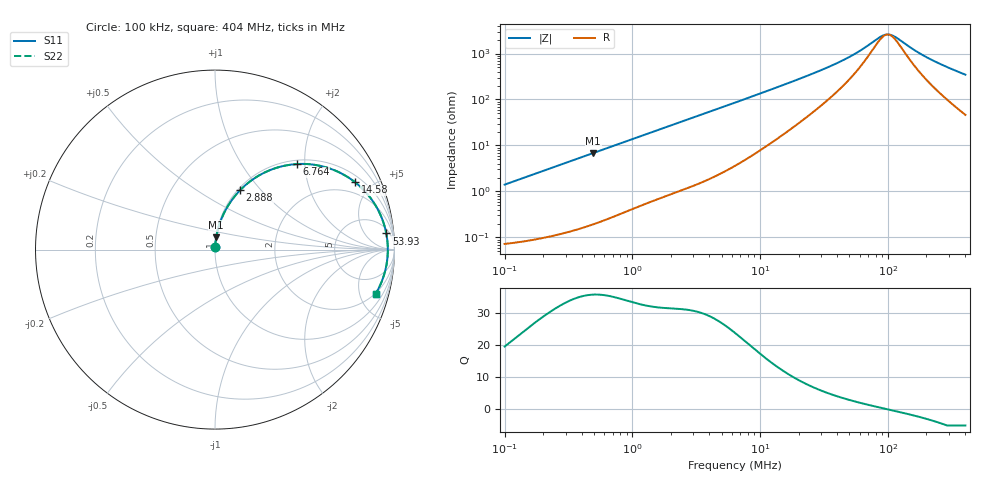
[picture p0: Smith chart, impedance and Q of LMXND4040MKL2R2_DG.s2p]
! LMXND4040MKL2R2_DG  S-PARAMETER MODEL  ( General Type )
! Model Generated by TAIYO YUDEN Corporation (http://www.ty-top.com)
! Version 1.0
! TAIYO YUDEN Control No. 191023NI43SB-FBB
! Copyright(c) 2019 TAIYO YUDEN CO.,LTD. All Rights Reserved.
! Product Description (link to TY-COMPAS)
! https://ds.yuden.co.jp/TYCOMPAS/or/detail?pn=LMXND4040MKL2R2MDG&u=M
! Products Name : Inductors
! Characteristics :
!  Inductance : 2.2 uH , SRF(min) : 70 MHz , DC Resistance(max) : 0.072 Ohm
!  Rated Current : Saturation :1650 mA , Temp Rise : 1900 mA
!  Case Size : 4.0 x 4.0 / 0.157 x 0.157 [mm/inch] , Thickness : 1.2 / 0.047 [mm/inch]
!  (Conditions: Temperature = 25 degC , DC Bias Current/Voltage = 0A / 0V)
! External Node Assignments :
!  1  o---GGG---o  2
! GND o---------o GND
! Frequency Range : 0.1MHz  -  403.964729MHz  [ 402 STEP ]
# MHz S RI R 50
! Freq[MHz].  S11 Real  S11 Imag  S21 Real  S21 Imag  S12 Real  S12 Imag  S22 Real  S22 Imag
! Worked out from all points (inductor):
!   401 points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, 100 kHz to 404 MHz, reference 50 ohm
!   read as one part in series: L = 2.23 uH near 104.2 kHz
!   highest Q = 35.6 at 494.6 kHz (marker M1), where L = 2.2 uH
!   self-resonance near 99.63 MHz
!   S11 on the Smith chart (normalised r, x): 100 kHz: 1.00, +0.03; 2.888 MHz: 1.03, +0.78; 6.764 MHz: 1.08, +1.82; 14.58 MHz: 1.32, +3.96; 53.93 MHz: 8, +18; 404 MHz: 1.92, -6.87
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0.1  0.000917 0.014  0.9991 -0.014  0.9991 -0.014  0.000917 0.014
0.401849  0.00467 0.0554  0.9953 -0.0554  0.9953 -0.0554  0.00467 0.0554
0.494562  0.00656 0.0679  0.9934 -0.0679  0.9934 -0.0679  0.00656 0.0679
0.921928  0.0193 0.1237  0.9807 -0.1237  0.9807 -0.1237  0.0193 0.1237
1.614823  0.0519 0.2066  0.9481 -0.2066  0.9481 -0.2066  0.0519 0.2066
2.887813  0.1394 0.3305  0.8606 -0.3305  0.8606 -0.3305  0.1394 0.3305
4.196184  0.2487 0.4151  0.7513 -0.4151  0.7513 -0.4151  0.2487 0.4151
6.355822  0.4247 0.4737  0.5753 -0.4737  0.5753 -0.4737  0.4247 0.4737
6.764245  0.4544 0.4765  0.5456 -0.4765  0.5456 -0.4765  0.4544 0.4765
9.626954  0.6209 0.4578  0.3791 -0.4578  0.3791 -0.4578  0.6209 0.4578
14.58163  0.7796 0.3761  0.2204 -0.3761  0.2204 -0.3761  0.7796 0.3761
25.54079  0.8999 0.237  0.1001 -0.237  0.1001 -0.237  0.8999 0.237
38.68579  0.9392 0.1485  0.0608 -0.1485  0.0608 -0.1485  0.9392 0.1485
53.92686  0.9543 0.0901  0.0457 -0.0901  0.0457 -0.0901  0.9543 0.0901
86.93005  0.9625 0.019  0.0375 -0.019  0.0375 -0.019  0.9625 0.019
94.45682  0.9629 0.00742  0.0371 -0.00742  0.0371 -0.00742  0.9629 0.00742
102.6353  0.9629 -0.00415  0.0371 0.00415  0.0371 0.00415  0.9629 -0.00415
116.2497  0.9625 -0.0216  0.0375 0.0216  0.0375 0.0216  0.9625 -0.0216
162.0487  0.9578 -0.0701  0.0422 0.0701  0.0422 0.0701  0.9578 -0.0701
207.8911  0.9501 -0.1105  0.0499 0.1105  0.0499 0.1105  0.9501 -0.1105
289.7942  0.9309 -0.1727  0.0691 0.1727  0.0691 0.1727  0.9309 -0.1727
403.9647  0.895 -0.2465  0.105 0.2465  0.105 0.2465  0.895 -0.2465
